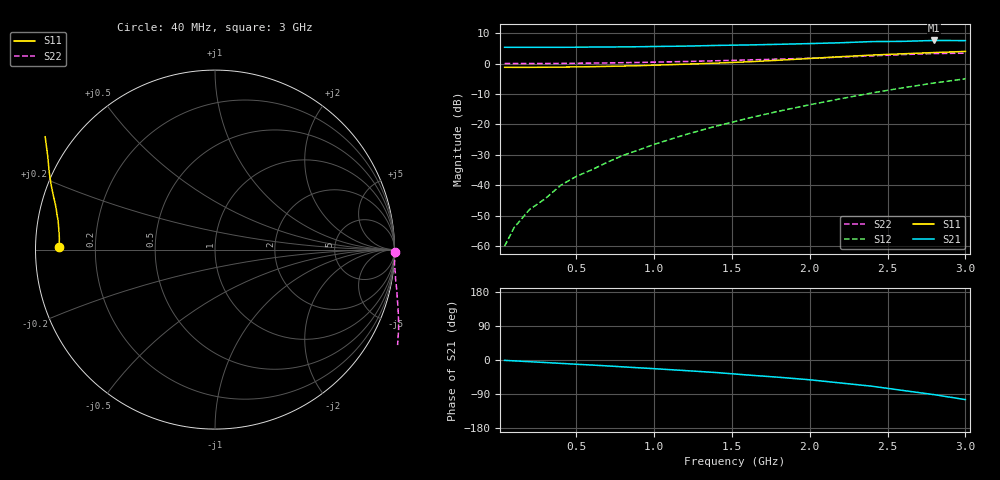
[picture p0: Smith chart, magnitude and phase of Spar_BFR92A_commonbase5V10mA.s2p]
! Filename:  BFR92ACC.S2P  Version:  2.0
! NXP part #: BFR92A  Date: Jul 1990
! Bias condition: Vce=5V, Ic=10mA
! COMMON BASE
#  MHz  S  MA  R  50
! Freq  S11  S21  S12  S22
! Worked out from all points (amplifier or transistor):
!   21 points, 40 MHz to 3 GHz, reference 50 ohm
!   highest |S21| = 7.6 dB at 2.8 GHz (marker M1)
!   |S21| within 3 dB of that: start of sweep to end of sweep
!   unconditionally stable (mu >= 1): nowhere
!   at 300 MHz: K = -0.54, MSG = 24.9 dB, |S12| = -44.4 dB
!   at 1 GHz: K = -0.94, MSG = 16.1 dB, |S12| = -26.6 dB
!   at 3 GHz: K = -0.87, MSG = 6.3 dB, |S12| = -5.0 dB
40  0.87 179.1  1.856 -1.0  0.001 47.7  1.002 -0.7
100  0.869 178.0  1.853 -2.2  0.002 75.1  1.004 -1.4
200  0.869 176.2  1.852 -4.5  0.004 110.8  1.003 -3.0
300  0.872 174.5  1.85 -6.6  0.006 120.0  1.003 -4.6
400  0.877 172.8  1.854 -8.9  0.01 130.5  1.008 -6.1
500  0.883 171.0  1.859 -11.2  0.014 134.7  1.014 -7.6
600  0.89 169.3  1.871 -13.3  0.018 138.8  1.019 -9.2
700  0.901 167.6  1.876 -15.6  0.024 141.3  1.027 -10.7
800  0.912 165.8  1.885 -18.1  0.031 143.2  1.036 -12.3
900  0.925 164.1  1.893 -20.5  0.038 145.2  1.046 -14.1
1000  0.942 162.3  1.912 -22.9  0.047 146.0  1.057 -15.8
1200  0.978 158.8  1.938 -27.9  0.068 146.8  1.083 -19.4
1400  1.019 155.0  1.99 -33.1  0.094 145.9  1.114 -23.3
1600  1.069 150.7  2.026 -39.6  0.126 145.1  1.148 -27.6
1800  1.136 146.4  2.075 -45.5  0.165 142.7  1.186 -32.5
2000  1.214 141.9  2.134 -52.2  0.211 139.7  1.226 -38.3
2200  1.3 137.2  2.202 -60.7  0.265 136.1  1.278 -45.2
2400  1.382 131.7  2.302 -69.2  0.33 131.2  1.342 -52.8
2600  1.45 124.7  2.322 -80.4  0.401 126.0  1.409 -61.2
2800  1.52 116.0  2.402 -91.5  0.481 119.1  1.464 -69.7
3000  1.585 106.6  2.386 -104.5  0.563 112.0  1.483 -79.5
